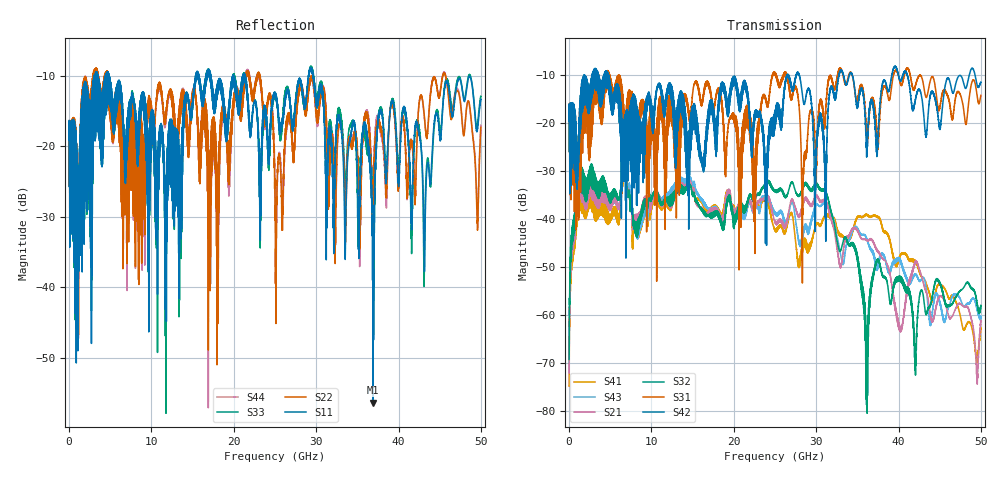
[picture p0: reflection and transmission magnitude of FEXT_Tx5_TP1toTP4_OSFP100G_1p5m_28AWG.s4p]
! Touchstone data
! Created: 27-Feb-2019 by IdEM 12 (12.1.0)
! COMMENTS
!  Created Wed Feb 27 09:43:39 2019
!  64 Port Network Data from SP1.SP block
!  freq  magS1_1  angS1_1  magS1_2  angS1_2  magS1_3  angS1_3  magS1_4  angS1_4
!  magS1_5  angS1_5  magS1_6  angS1_6  magS1_7  angS1_7  magS1_8  angS1_8
!  magS1_9  angS1_9  magS1_10  angS1_10  magS1_11  angS1_11  magS1_12  angS1_12
!  magS1_13  angS1_13  magS1_14  angS1_14  magS1_15  angS1_15  magS1_16  angS1_16
!  magS1_17  angS1_17  magS1_18  angS1_18  magS1_19  angS1_19  magS1_20  angS1_20
!  magS1_21  angS1_21  magS1_22  angS1_22  magS1_23  angS1_23  magS1_24  angS1_24
!  magS1_25  angS1_25  magS1_26  angS1_26  magS1_27  angS1_27  magS1_28  angS1_28
!  magS1_29  angS1_29  magS1_30  angS1_30  magS1_31  angS1_31  magS1_32  angS1_32
!  magS1_33  angS1_33  magS1_34  angS1_34  magS1_35  angS1_35  magS1_36  angS1_36
!  magS1_37  angS1_37  magS1_38  angS1_38  magS1_39  angS1_39  magS1_40  angS1_40
!  magS1_41  angS1_41  magS1_42  angS1_42  magS1_43  angS1_43  magS1_44  angS1_44
!  magS1_45  angS1_45  magS1_46  angS1_46  magS1_47  angS1_47  magS1_48  angS1_48
!  magS1_49  angS1_49  magS1_50  angS1_50  magS1_51  angS1_51  magS1_52  angS1_52
!  magS1_53  angS1_53  magS1_54  angS1_54  magS1_55  angS1_55  magS1_56  angS1_56
!  magS1_57  angS1_57  magS1_58  angS1_58  magS1_59  angS1_59  magS1_60  angS1_60
!  magS1_61  angS1_61  magS1_62  angS1_62  magS1_63  angS1_63  magS1_64  angS1_64
!  magS2_1  angS2_1  magS2_2  angS2_2  magS2_3  angS2_3  magS2_4  angS2_4
!  magS2_5  angS2_5  magS2_6  angS2_6  magS2_7  angS2_7  magS2_8  angS2_8
!  magS2_9  angS2_9  magS2_10  angS2_10  magS2_11  angS2_11  magS2_12  angS2_12
!  magS2_13  angS2_13  magS2_14  angS2_14  magS2_15  angS2_15  magS2_16  angS2_16
!  magS2_17  angS2_17  magS2_18  angS2_18  magS2_19  angS2_19  magS2_20  angS2_20
!  magS2_21  angS2_21  magS2_22  angS2_22  magS2_23  angS2_23  magS2_24  angS2_24
!  magS2_25  angS2_25  magS2_26  angS2_26  magS2_27  angS2_27  magS2_28  angS2_28
!  magS2_29  angS2_29  magS2_30  angS2_30  magS2_31  angS2_31  magS2_32  angS2_32
!  magS2_33  angS2_33  magS2_34  angS2_34  magS2_35  angS2_35  magS2_36  angS2_36
!  magS2_37  angS2_37  magS2_38  angS2_38  magS2_39  angS2_39  magS2_40  angS2_40
!  magS2_41  angS2_41  magS2_42  angS2_42  magS2_43  angS2_43  magS2_44  angS2_44
!  magS2_45  angS2_45  magS2_46  angS2_46  magS2_47  angS2_47  magS2_48  angS2_48
!  magS2_49  angS2_49  magS2_50  angS2_50  magS2_51  angS2_51  magS2_52  angS2_52
!  magS2_53  angS2_53  magS2_54  angS2_54  magS2_55  angS2_55  magS2_56  angS2_56
!  magS2_57  angS2_57  magS2_58  angS2_58  magS2_59  angS2_59  magS2_60  angS2_60
!  magS2_61  angS2_61  magS2_62  angS2_62  magS2_63  angS2_63  magS2_64  angS2_64
!  magS3_1  angS3_1  magS3_2  angS3_2  magS3_3  angS3_3  magS3_4  angS3_4
!  magS3_5  angS3_5  magS3_6  angS3_6  magS3_7  angS3_7  magS3_8  angS3_8
!  magS3_9  angS3_9  magS3_10  angS3_10  magS3_11  angS3_11  magS3_12  angS3_12
!  magS3_13  angS3_13  magS3_14  angS3_14  magS3_15  angS3_15  magS3_16  angS3_16
!  magS3_17  angS3_17  magS3_18  angS3_18  magS3_19  angS3_19  magS3_20  angS3_20
!  magS3_21  angS3_21  magS3_22  angS3_22  magS3_23  angS3_23  magS3_24  angS3_24
!  magS3_25  angS3_25  magS3_26  angS3_26  magS3_27  angS3_27  magS3_28  angS3_28
!  magS3_29  angS3_29  magS3_30  angS3_30  magS3_31  angS3_31  magS3_32  angS3_32
!  magS3_33  angS3_33  magS3_34  angS3_34  magS3_35  angS3_35  magS3_36  angS3_36
!  magS3_37  angS3_37  magS3_38  angS3_38  magS3_39  angS3_39  magS3_40  angS3_40
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# Hz S MA R 50
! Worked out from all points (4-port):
!   5000 points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, 10 MHz to 50 GHz, reference 50 ohm
!   strongest paths, dB at 10 MHz, 12.51 GHz, 25.01 GHz, 37.51 GHz, 50 GHz:
!     S42: -19.6, -13.5, -17.4, -23.0, -11.4
!     S31: -19.6, -16.6, -9.8, -25.4, -14.2
!     S32: -69.2, -36.1, -34.0, -48.3, -58.1
!     S21: -72.0, -35.9, -40.6, -46.7, -61.3
!     S43: -71.9, -34.4, -38.5, -49.2, -60.6
!     S41: -74.8, -35.5, -42.3, -39.4, -62.9
!   lowest |S11| = -56.3 dB at 36.9 GHz (marker M1), VSWR 1.00, Z = 50.1 + j0.121 ohm
!   |S11| at or under -10 dB: 4.861 GHz to 15.4 GHz (10.54 GHz wide, 104 % of centre); 21.38 GHz to 29.07 GHz (7.682 GHz wide, 30.5 % of centre); 29.66 GHz to end of sweep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
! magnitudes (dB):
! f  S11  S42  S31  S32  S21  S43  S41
! 10 MHz  -19.1  -19.6  -19.6  -69.2  -72.0  -71.9  -74.8
! 1.36 GHz  -23.2  -19.1  -21.7  -30.0  -31.8  -31.7  -33.8
! 6.73 GHz  -19.4  -21.0  -18.9  -28.8  -29.2  -29.1  -29.8
! 29.37 GHz  -8.8  -15.2  -17.4  -34.2  -37.3  -40.9  -45.1
! 36.11 GHz  -17.8  -24.9  -22.1  -68.8  -44.4  -44.0  -39.0
! 36.9 GHz  -56.3  -15.8  -14.9  -52.3  -44.8  -47.3  -39.3
! 50 GHz  -13.4  -11.4  -14.2  -58.1  -61.3  -60.6  -62.9
